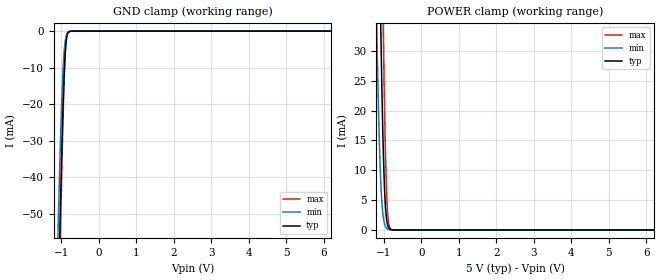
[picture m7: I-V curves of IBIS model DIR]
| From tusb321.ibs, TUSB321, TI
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|   Model
[Model]   DIR
Model_type   Input
Vinl = 1.5
Vinh = 3.5
|   typ   min   max
C_comp   0.453pF   0.401pF   0.510pF
[Voltage Range]   5   4.999   5.001
[Temperature Range]   27   105   -40
[Power Clamp Reference]   5   4.999   5.001
[GND Clamp Reference]   0   0   0
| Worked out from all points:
|   GND clamp passes 1 mA (typ) near -0.84 V on its own axis
|   POWER clamp passes 1 mA (typ) near -0.90 V on its own axis
[GND Clamp]
|   Voltage   I(typ)   I(min)   I(max)
-5V       -2.267A    -2.153A    -2.357A
-1.1V     -83.39mA   -59.91mA   -94.16mA
-1.085V   -76.15mA   -53.61mA   -86.34mA
-1.04V    -55.17mA   -35.94mA   -63.45mA
-1.025V   -48.5mA    -30.57mA   -56.07mA
-965mV    -24.37mA   -12.92mA   -28.65mA
-935mV    -14.7mA    -7.113mA   -17.09mA
-905mV    -7.501mA   -3.473mA   -8.164mA
-890mV    -4.983mA   -2.337mA   -5.042mA
-860mV    -1.926mA   -1.006mA   -1.531mA
-815mV    -380.4uA   -267.2uA   -188.9uA
10V       0A         0A         0A
[POWER Clamp]
|   Voltage   I(typ)   I(min)   I(max)
-5V       2.317A     2.221A     2.385A
-1.19V    81.55mA    34.73mA    119mA
-1.13V    53.92mA    17.14mA    87.53mA
-1.085V   35.47mA    8.494mA    65.05mA
-1.025V   15.94mA    2.68mA     37.58mA
-1.01V    12.3mA     1.954mA    31.4mA
-980mV    6.741mA    1.018mA    20.31mA
-935mV    2.276mA    372.6uA    8.066mA
-905mV    1.017mA    189uA      3.499mA
-875mV    440uA      95.65uA    1.312mA
-710mV    4.408uA    2.676uA    3.805uA
10V       0A         0A         0A
